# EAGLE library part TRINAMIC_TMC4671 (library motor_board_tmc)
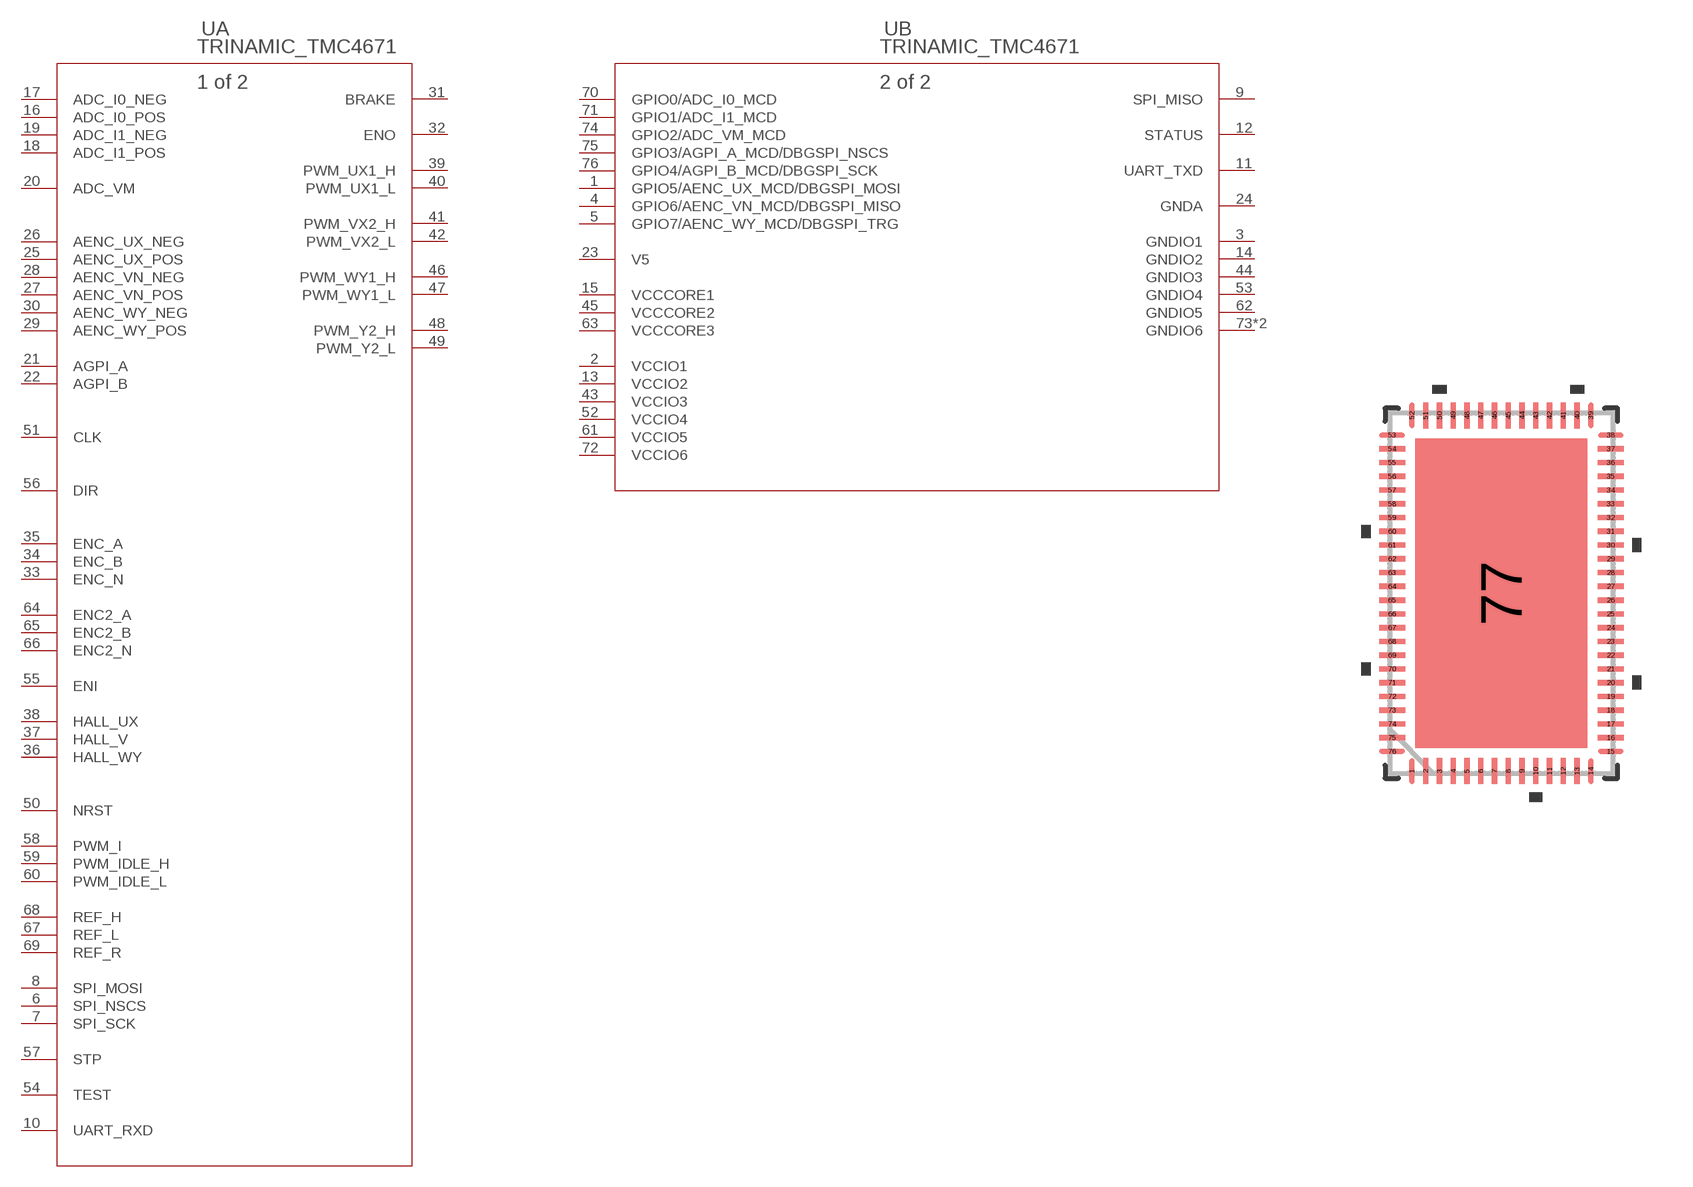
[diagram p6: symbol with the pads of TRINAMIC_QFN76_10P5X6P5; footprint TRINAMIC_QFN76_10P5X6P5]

Designator prefix U; gates A=TRINAMIC_TMC4671-ES B=TRINAMIC_TMC4671-ES_A

## TRINAMIC_TMC4671 (MANUFACTURER_PART_NUMBER: TMC4671ES; VENDOR: TRINAMIC)  [TRINAMIC_QFN76_10P5X6P5]
1  B:GPIO5/AENC_UX_MCD/DBGSPI_MOSI
2  B:VCCIO1  pwr
3  B:GNDIO1  pwr
4  B:GPIO6/AENC_VN_MCD/DBGSPI_MISO
5  B:GPIO7/AENC_WY_MCD/DBGSPI_TRG
6  A:SPI_NSCS  in
7  A:SPI_SCK  in
8  A:SPI_MOSI  in
9  B:SPI_MISO  out
10  A:UART_RXD  in
11  B:UART_TXD  out
12  B:STATUS  out
13  B:VCCIO2  pwr
14  B:GNDIO2  pwr
15  B:VCCCORE1  pwr
16  A:ADC_I0_POS  in
17  A:ADC_I0_NEG  in
18  A:ADC_I1_POS  in
19  A:ADC_I1_NEG  in
20  A:ADC_VM  in
21  A:AGPI_A  in
22  A:AGPI_B  in
23  B:V5  pwr
24  B:GNDA  pwr
25  A:AENC_UX_POS  in
26  A:AENC_UX_NEG  in
27  A:AENC_VN_POS  in
28  A:AENC_VN_NEG  in
29  A:AENC_WY_POS  in
30  A:AENC_WY_NEG  in
31  A:BRAKE  out
32  A:ENO  out
33  A:ENC_N  in
34  A:ENC_B  in
35  A:ENC_A  in
36  A:HALL_WY  in
37  A:HALL_V  in
38  A:HALL_UX  in
39  A:PWM_UX1_H  out
40  A:PWM_UX1_L  out
41  A:PWM_VX2_H  out
42  A:PWM_VX2_L  out
43  B:VCCIO3  pwr
44  B:GNDIO3  pwr
45  B:VCCCORE2  pwr
46  A:PWM_WY1_H  out
47  A:PWM_WY1_L  out
48  A:PWM_Y2_H  out
49  A:PWM_Y2_L  out
50  A:NRST  in
51  A:CLK  in
52  B:VCCIO4  pwr
53  B:GNDIO4  pwr
54  A:TEST  in
55  A:ENI  in
56  A:DIR  in
57  A:STP  in
58  A:PWM_I  in
59  A:PWM_IDLE_H  in
60  A:PWM_IDLE_L  in
61  B:VCCIO5  pwr
62  B:GNDIO5  pwr
63  B:VCCCORE3  pwr
64  A:ENC2_A  in
65  A:ENC2_B  in
66  A:ENC2_N  in
67  A:REF_L  in
68  A:REF_H  in
69  A:REF_R  in
70  B:GPIO0/ADC_I0_MCD
71  B:GPIO1/ADC_I1_MCD
72  B:VCCIO6  pwr
73  B:GNDIO6  pwr
74  B:GPIO2/ADC_VM_MCD
75  B:GPIO3/AGPI_A_MCD/DBGSPI_NSCS
76  B:GPIO4/AGPI_B_MCD/DBGSPI_SCK
77  B:GNDIO6  pwr

## Footprint TRINAMIC_QFN76_10P5X6P5 (pad centres in mm)
smd 0.152 x 0.755: 1 -2.6,-5.173; 2 -2.2,-5.173; 3 -1.8,-5.173; 4 -1.4,-5.173; 5 -1,-5.173; 6 -0.6,-5.173; 7 -0.2,-5.173; 8 0.2,-5.173; 9 0.6,-5.173; 10 1,-5.173; 11 1.4,-5.173; 12 1.8,-5.173; 13 2.2,-5.173; 14 2.6,-5.173; 39 2.6,5.173; 40 2.2,5.173; 41 1.8,5.173; 42 1.4,5.173; 43 1,5.173; 44 0.6,5.173; 45 0.2,5.173; 46 -0.2,5.173; 47 -0.6,5.173; 48 -1,5.173; 49 -1.4,5.173; 50 -1.8,5.173; 51 -2.2,5.173; 52 -2.6,5.173
smd 0.755 x 0.152: 15 3.179,-4.6; 16 3.179,-4.2; 17 3.179,-3.8; 18 3.179,-3.4; 19 3.179,-3; 20 3.179,-2.6; 21 3.179,-2.2; 22 3.179,-1.8; 23 3.179,-1.4; 24 3.179,-1; 25 3.179,-0.6; 26 3.179,-0.2; 27 3.179,0.2; 28 3.179,0.6; 29 3.179,1; 30 3.179,1.4; 31 3.179,1.8; 32 3.179,2.2; 33 3.179,2.6; 34 3.179,3; 35 3.179,3.4; 36 3.179,3.8; 37 3.179,4.2; 38 3.179,4.6; 53 -3.179,4.6; 54 -3.179,4.2; 55 -3.179,3.8; 56 -3.179,3.4; 57 -3.179,3; 58 -3.179,2.6; 59 -3.179,2.2; 60 -3.179,1.8; 61 -3.179,1.4; 62 -3.179,1; 63 -3.179,0.6; 64 -3.179,0.2; 65 -3.179,-0.2; 66 -3.179,-0.6; 67 -3.179,-1; 68 -3.179,-1.4; 69 -3.179,-1.8; 70 -3.179,-2.2; 71 -3.179,-2.6; 72 -3.179,-3; 73 -3.179,-3.4; 74 -3.179,-3.8; 75 -3.179,-4.2; 76 -3.179,-4.6
smd 5.004 x 8.992: 77 0,0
